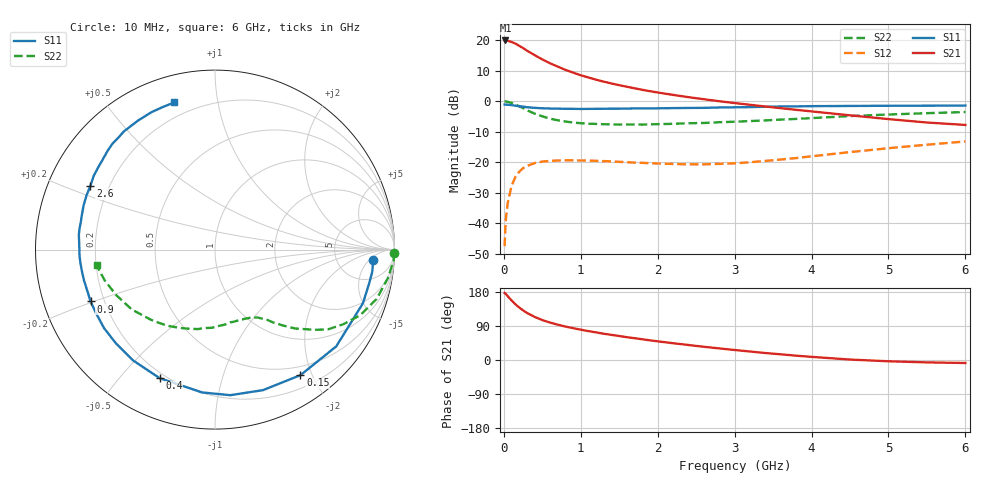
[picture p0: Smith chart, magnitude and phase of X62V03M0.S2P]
! SIEMENS Small Signal Semiconductors
! BFP193W
! Si NPN RF Bipolar Junction Transistor in SOT343
! VCE = 2 V  IC = 3 mA
! Common Emitter S-Parameters:  April 1994
# GHz  S  MA  R  50
!  f  S11  S21  S12  S22
! GHz  MAG  ANG  MAG  ANG  MAG  ANG  MAG  ANG
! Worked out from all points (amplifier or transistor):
!   40 points, 10 MHz to 6 GHz, reference 50 ohm
!   highest |S21| = 19.9 dB at 20 MHz (marker M1)
!   |S21| within 3 dB of that: start of sweep to 280.7 MHz
!   unconditionally stable (mu >= 1): 1.894 GHz to 4.854 GHz
!   at 200 MHz: K = 0.10, MSG = 20.7 dB, |S12| = -23.1 dB
!   at 1.5 GHz: K = 0.79, MSG = 12.6 dB, |S12| = -19.9 dB
!   at 6 GHz: K = 0.96, MSG = 2.7 dB, |S12| = -13.2 dB
!   S11 on the Smith chart (normalised r, x): 10 MHz: 12, -7; 150 MHz: 0.37, -1.83; 400 MHz: 0.18, -0.64; 900 MHz: 0.15, -0.20; 2.6 GHz: 0.13, +0.24; 6 GHz: 0.13, +0.75
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0.01  0.8837 -3.9  9.888 176.9  0.0042 87.6  0.9997 -1.0
0.02  0.8847 -8.0  9.938 175.4  0.0086 84.2  0.9964 -3.7
0.05  0.8769 -19.9  9.819 168.5  0.0213 79.3  0.9789 -8.9
0.1  0.8643 -38.6  9.395 157.4  0.0406 69.3  0.9416 -17.0
0.15  0.8462 -55.8  8.824 147.2  0.0573 60.5  0.887 -24.4
0.2  0.8275 -71.1  8.116 138.4  0.0698 53.2  0.8269 -30.2
0.25  0.8156 -84.0  7.459 131.0  0.0798 46.5  0.7698 -35.3
0.3  0.799 -95.2  6.782 124.3  0.0869 41.3  0.7133 -38.8
0.4  0.7799 -113.3  5.707 113.8  0.0967 33.1  0.6273 -44.5
0.5  0.7678 -126.5  4.86 105.4  0.1024 27.4  0.5655 -48.3
0.6  0.7598 -136.7  4.2 98.8  0.1051 22.8  0.5195 -51.4
0.7  0.7572 -144.8  3.705 93.3  0.1068 19.9  0.4875 -53.4
0.9  0.7509 -157.4  2.952 84.0  0.1075 15.3  0.4482 -57.7
1.1  0.7498 -166.7  2.455 76.2  0.1064 12.5  0.4277 -61.9
1.3  0.7534 -174.2  2.095 69.3  0.1044 10.9  0.4199 -66.4
1.6  0.7585 176.5  1.73 60.2  0.1002 10.7  0.415 -73.0
2.2  0.7725 161.5  1.272 44.3  0.0936 15.2  0.4263 -87.5
2.6  0.7796 152.9  1.08 34.9  0.0924 21.3  0.4406 -97.5
3.2  0.8019 141.3  0.876 22.4  0.0998 31.3  0.4734 -112.2
4.5  0.8373 120.7  0.588 1.2  0.1467 41.4  0.5714 -144.3
5.5  0.8455 110.5  0.448 -6.3  0.1938 39.1  0.638 -164.4
6  0.8509 105.4  0.409 -7.9  0.2191 37.0  0.6656 -172.4
